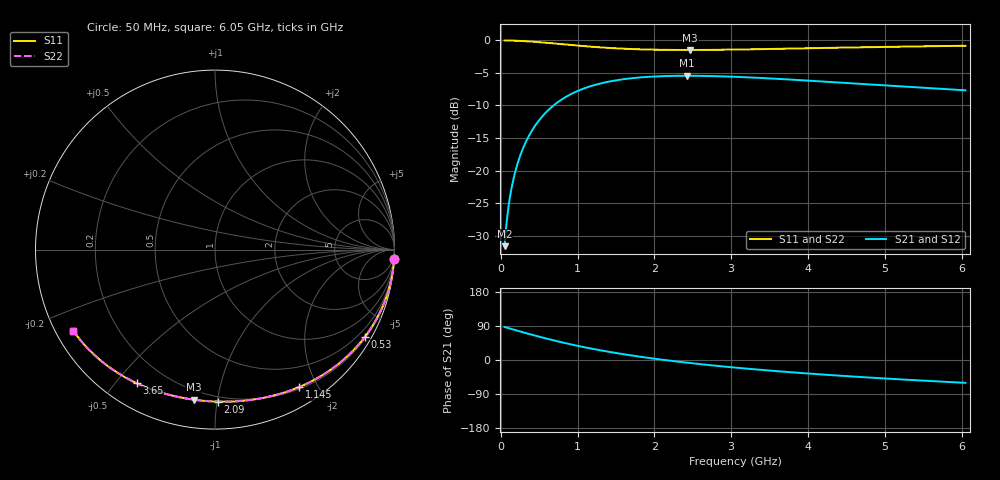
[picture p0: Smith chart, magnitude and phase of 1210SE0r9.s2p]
! AVX Thin Film Operation		Date: August 2001
! Description: Accu-P® Series, Thin Film, SMD, RF Capacitor
! Part Number: 12101J0R9ABT
! 50 MHz  -  6.05 GHz
! Serial Measurements
# mhz S db R 50
!	S11		S21		S12		S22
!	dB	Phase	dB	Phase	dB	Phase	dB	Phase
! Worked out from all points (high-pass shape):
!   401 points, 50 MHz to 6.05 GHz, reference 50 ohm
!   highest |S21| = -5.43 dB at 2.42 GHz (marker M1); lowest = -31.6 dB at 50 MHz (marker M2)
!   |S21| within 3 dB of the highest: 885.8 MHz to end of sweep
!   lowest |S11| = -1.5 dB at 2.465 GHz (marker M3), VSWR 11.86, Z = 7.36 - j42.9 ohm
!   |S11| at or under -10 dB: nowhere
!   |S22| runs from -1.5 to 0.0 dB; largest |S21 - S12| = 0
!   S11 on the Smith chart (normalised r, x): 50 MHz: 0, -39; 530 MHz: 0.25, -3.70; 1.145 GHz: 0.22, -1.76; 2.09 GHz: 0.17, -1.01; 3.65 GHz: 0.10, -0.57; 6.05 GHz: 0.05, -0.27
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50  -0.00 -2.9  -31.64 87.1  -31.64 87.1  -0.00 -2.9
65  -0.01 -3.8  -29.36 86.2  -29.36 86.2  -0.01 -3.8
125  -0.02 -7.4  -23.71 82.7  -23.71 82.7  -0.02 -7.4
170  -0.03 -10.0  -21.08 80.0  -21.08 80.0  -0.03 -10.0
215  -0.05 -12.6  -19.08 77.4  -19.08 77.4  -0.05 -12.6
275  -0.09 -16.0  -17.02 74.0  -17.02 74.0  -0.09 -16.0
350  -0.14 -20.3  -15.05 69.7  -15.05 69.7  -0.14 -20.3
440  -0.21 -25.3  -13.23 64.7  -13.23 64.7  -0.21 -25.3
530  -0.29 -30.1  -11.83 59.9  -11.83 59.9  -0.29 -30.1
770  -0.55 -42.2  -9.27 47.8  -9.27 47.8  -0.55 -42.2
1055  -0.85 -54.9  -7.51 35.1  -7.51 35.1  -0.85 -54.9
1145  -0.94 -58.6  -7.13 31.4  -7.13 31.4  -0.94 -58.6
1580  -1.26 -74.2  -5.99 15.8  -5.99 15.8  -1.26 -74.2
2060  -1.44 -88.1  -5.51 1.9  -5.51 1.9  -1.44 -88.1
2090  -1.44 -88.9  -5.50 1.1  -5.50 1.1  -1.44 -88.9
2420  -1.47 -97.0  -5.43 -7.0  -5.43 -7.0  -1.47 -96.9
2465  -1.47 -98.0  -5.43 -8.0  -5.43 -8.0  -1.47 -98.0
3050  -1.41 -110.0  -5.59 -20.0  -5.59 -20.0  -1.41 -110.0
3650  -1.28 -120.3  -5.93 -30.3  -5.93 -30.3  -1.28 -120.3
4055  -1.19 -126.4  -6.22 -36.4  -6.22 -36.4  -1.19 -126.4
5060  -0.98 -139.4  -6.97 -49.5  -6.97 -49.5  -0.98 -139.4
6050  -0.82 -150.2  -7.67 -60.3  -7.67 -60.3  -0.82 -150.2
